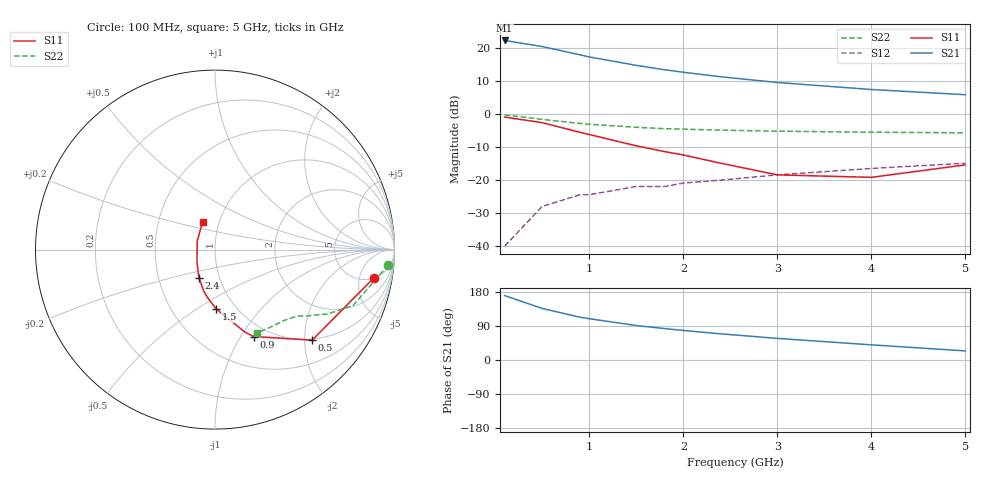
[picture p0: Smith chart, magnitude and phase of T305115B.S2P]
!AT-30511
!S and NOISE PARAMETERS at Vce=5V  Ic=5mA.  LAST UPDATED 04-10-94
# ghz s ma r 50
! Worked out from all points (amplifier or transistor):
!   11 points, 100 MHz to 5 GHz, reference 50 ohm
!   highest |S21| = 22.3 dB at 100 MHz (marker M1)
!   |S21| within 3 dB of that: start of sweep to 685.1 MHz
!   unconditionally stable (mu >= 1): 2.114 GHz to end of sweep
!   at 500 MHz: K = 0.41, MSG = 24.2 dB, |S12| = -28.0 dB
!   at 1.8 GHz: K = 0.97, MSG = 17.7 dB, |S12| = -21.9 dB
!   at 5 GHz: K = 1.09, MAG = 8.5 dB, |S12| = -14.9 dB
!   lowest NFmin = 1.10 dB at 500 MHz
!   S11 on the Smith chart (normalised r, x): 100 MHz: 5.09, -8.37; 500 MHz: 0.97, -2.17; 900 MHz: 0.85, -1.14; 1.5 GHz: 0.81, -0.60; 2.4 GHz: 0.80, -0.26; 5 GHz: 0.83, +0.27
0.1  0.9 -10.0  12.98 170.0  0.01 82.0  0.97 -5.0
0.5  0.74 -43.0  10.49 136.0  0.04 66.0  0.83 -22.0
0.9  0.53 -66.0  7.88 113.0  0.06 58.0  0.72 -30.0
1  0.49 -70.0  7.31 109.0  0.06 57.0  0.7 -31.0
1.5  0.33 -89.0  5.45 91.0  0.08 54.0  0.63 -36.0
1.8  0.27 -99.0  4.68 83.0  0.08 53.0  0.6 -38.0
2  0.24 -105.0  4.29 78.0  0.09 52.0  0.59 -39.0
2.4  0.18 -120.0  3.66 69.0  0.1 50.0  0.57 -42.0
3  0.12 -147.0  3 57.0  0.12 48.0  0.55 -46.0
4  0.11 154.0  2.35 40.0  0.15 43.0  0.53 -55.0
5  0.17 114.0  1.96 24.0  0.18 38.0  0.52 -63.0
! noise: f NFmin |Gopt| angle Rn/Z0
0.5  1.1  0.77  9  1.1
0.9  1.2  0.71  18  0.96
1.8  1.5  0.6  45  0.66
2.4  1.8  0.51  65  0.47
